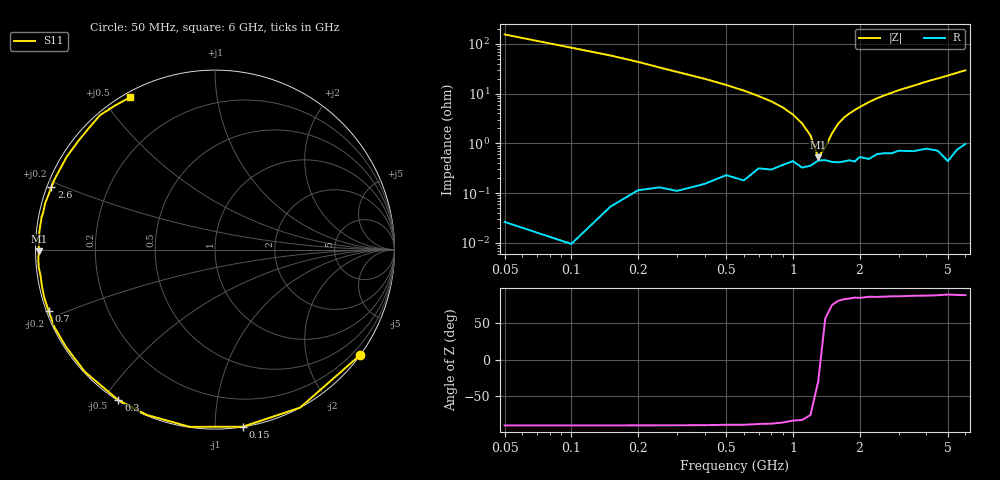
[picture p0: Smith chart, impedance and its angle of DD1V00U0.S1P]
! Infineon Technologies  Discrete & RF Semiconductors
! BBY58-02W
! Si Tuning Diode in SCD-80
! VR = 1 V
! S-Parameters:  June  2000
# GHz  S  MA  R  50
!  f  S11
! GHz  MAG  ANG
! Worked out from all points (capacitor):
!   34 points, 50 MHz to 6 GHz, reference 50 ohm
!   read as one part to ground: C = 18.9 pF near 50 MHz
!   lowest |Z| = 522 mohm at 1.3 GHz (marker M1)
!   series resonance near 1.327 GHz, so ESL is about 760 pH
!   S11 on the Smith chart (normalised r, x): 50 MHz: 0.00, -3.09; 150 MHz: 0.00, -1.17; 300 MHz: 0.00, -0.55; 700 MHz: 0.01, -0.18; 2.6 GHz: 0.01, +0.19; 6 GHz: 0.02, +0.59
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0.05  0.9999 -35.9
0.1  0.9999 -61.7
0.15  0.9991 -81.1
0.2  0.9974 -98.1
0.25  0.9964 -112.4
0.3  0.9966 -122.7
0.4  0.9947 -136.8
0.5  0.9916 -146.8
0.6  0.9932 -154.1
0.7  0.9879 -159.8
0.8  0.9884 -164.2
0.9  0.9855 -168.0
1  0.9827 -171.4
1.1  0.9871 -174.3
1.3  0.9821 -179.4
1.6  0.9836 174.4
1.7  0.9829 172.5
1.9  0.9831 169.4
2  0.9792 167.8
2.2  0.9811 164.7
2.4  0.9765 161.7
2.6  0.9758 159.0
3  0.9734 153.7
3.5  0.9746 147.9
4  0.9725 141.6
5  0.9856 130.5
5.5  0.9769 124.7
6  0.9714 119.1
